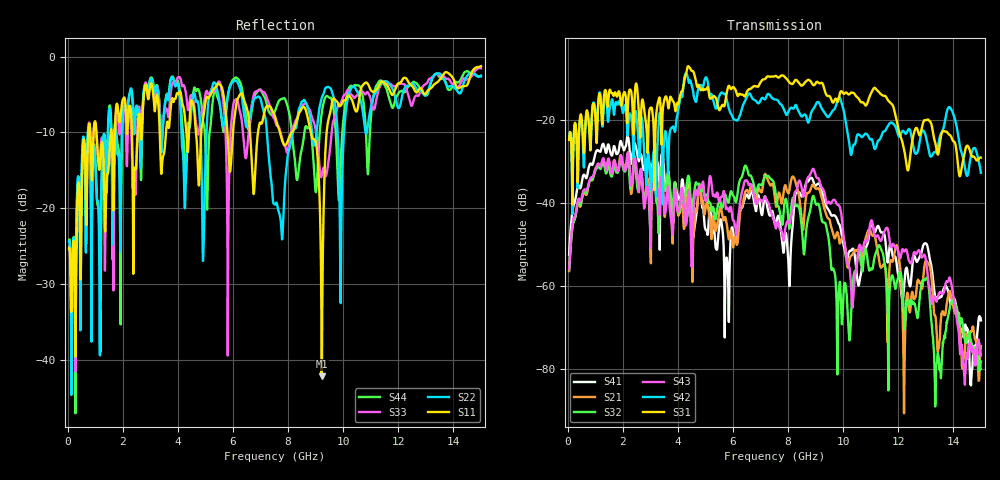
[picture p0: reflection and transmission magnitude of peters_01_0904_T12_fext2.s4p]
# MHZ S RI R 50.00
! FREQ  S11  S12  S13  S14
!  S21  S22  S23  S24
!  S31  S32  S33  S34
!  S41  S42  S43  S44
!  REAL  IMAG  REAL  IMAG  REAL  IMAG  REAL  IMAG
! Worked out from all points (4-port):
!   1496 points, 50 MHz to 15 GHz, reference 50 ohm
!   strongest paths, dB at 50 MHz, 3.79 GHz, 7.53 GHz, 11.27 GHz, 15 GHz:
!     S31: -24.9, -15.3, -9.5, -13.2, -29.1
!     S42: -24.8, -21.9, -15.2, -25.1, -32.8
!     S43: -56.0, -46.5, -45.4, -47.9, -76.5
!     S32: -56.2, -42.6, -36.8, -50.5, -78.2
!     S21: -56.4, -47.4, -39.4, -52.3, -74.5
!     S41: -52.5, -40.4, -45.4, -45.6, -68.3
!   lowest |S11| = -42.1 dB at 9.22 GHz (marker M1), VSWR 1.02, Z = 50.8 - j0.157 ohm
!   |S11| at or under -10 dB: start of sweep to 747.8 MHz; 1.045 GHz to 1.556 GHz (511.3 MHz wide, 39.3 % of centre); 8.823 GHz to 9.399 GHz (575.5 MHz wide, 6.32 % of centre)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
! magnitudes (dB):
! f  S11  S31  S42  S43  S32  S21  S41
! 50 MHz  -25.3  -24.9  -24.8  -56.0  -56.2  -56.4  -52.5
! 2.16 GHz  -10.2  -20.9  -22.9  -28.5  -29.5  -28.6  -24.1
! 5.49 GHz  -3.6  -17.6  -14.5  -39.6  -39.9  -42.8  -46.6
! 9.22 GHz  -42.1  -11.2  -17.3  -36.3  -44.2  -38.7  -37.2
! 9.65 GHz  -5.5  -15.9  -17.7  -39.3  -56.1  -47.8  -43.0
! 10.34 GHz  -5.9  -13.6  -27.0  -65.2  -60.4  -52.4  -51.1
! 15 GHz  -1.3  -29.1  -32.8  -76.5  -78.2  -74.5  -68.3
